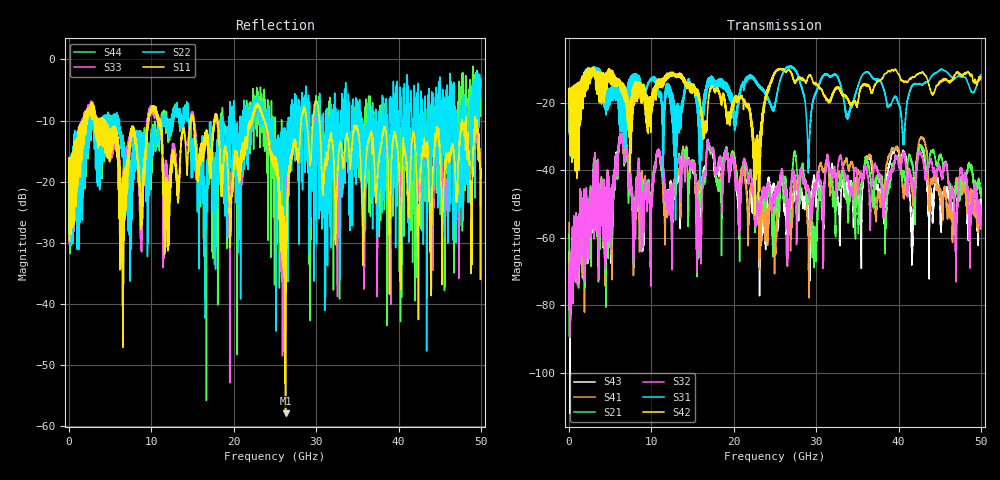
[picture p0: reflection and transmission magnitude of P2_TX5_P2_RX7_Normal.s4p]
!Keysight Technologies,N5225B,MY57041031,A.13.20.10
!Date: Friday, May 31, 2019 11:37:56
!Correction: S11(Full 4 Port(1,2,3,4))
!S12(Full 4 Port(1,2,3,4))
!S13(Full 4 Port(1,2,3,4))
!S14(Full 4 Port(1,2,3,4))
!S21(Full 4 Port(1,2,3,4))
!S22(Full 4 Port(1,2,3,4))
!S23(Full 4 Port(1,2,3,4))
!S24(Full 4 Port(1,2,3,4))
!S31(Full 4 Port(1,2,3,4))
!S32(Full 4 Port(1,2,3,4))
!S33(Full 4 Port(1,2,3,4))
!S34(Full 4 Port(1,2,3,4))
!S41(Full 4 Port(1,2,3,4))
!S42(Full 4 Port(1,2,3,4))
!S43(Full 4 Port(1,2,3,4))
!S44(Full 4 Port(1,2,3,4))
!S4P File: Measurements: <S11,S12,S13,S14>,
!<S21,S22,S23,S24>,
!<S31,S32,S33,S34>,
!<S41,S42,S43,S44>:
# Hz S  dB  R 50.0
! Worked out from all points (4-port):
!   5000 points, 10 MHz to 50 GHz, reference 50 ohm
!   strongest paths, dB at 10 MHz, 12.51 GHz, 25.01 GHz, 37.51 GHz, 50 GHz:
!     S42: -19.5, -12.0, -11.4, -13.5, -12.3
!     S31: -19.3, -17.8, -20.9, -13.2, -11.7
!     S32: -67.5, -52.3, -47.0, -40.7, -55.2
!     S21: -58.8, -52.5, -51.5, -42.0, -45.2
!     S41: -55.5, -53.9, -60.6, -46.4, -53.0
!     S43: -68.5, -59.3, -46.2, -44.5, -48.3
!   lowest |S11| = -57.9 dB at 26.29 GHz (marker M1), VSWR 1.00, Z = 50.1 - j0.0107 ohm
!   |S11| at or under -10 dB: 4.282 GHz to 9.568 GHz (5.286 GHz wide, 76.3 % of centre); 23.74 GHz to 28.18 GHz (4.44 GHz wide, 17.1 % of centre); 30.41 GHz to 47.71 GHz (17.3 GHz wide, 44.3 % of centre)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
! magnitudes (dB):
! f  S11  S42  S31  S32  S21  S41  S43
! 10 MHz  -19.8  -19.5  -19.3  -67.5  -58.8  -55.5  -68.5
! 6.28 GHz  -21.7  -13.9  -24.9  -30.9  -31.2  -30.7  -30.4
! 7.87 GHz  -11.7  -14.8  -12.2  -66.1  -59.6  -60.4  -68.8
! 22.8 GHz  -7.6  -37.0  -14.3  -49.4  -48.5  -51.2  -51.4
! 26.29 GHz  -57.9  -11.0  -9.7  -45.2  -42.1  -47.4  -51.3
! 30.01 GHz  -6.8  -14.6  -16.7  -44.3  -61.2  -44.3  -47.5
! 50 GHz  -19.3  -12.3  -11.7  -55.2  -45.2  -53.0  -48.3
